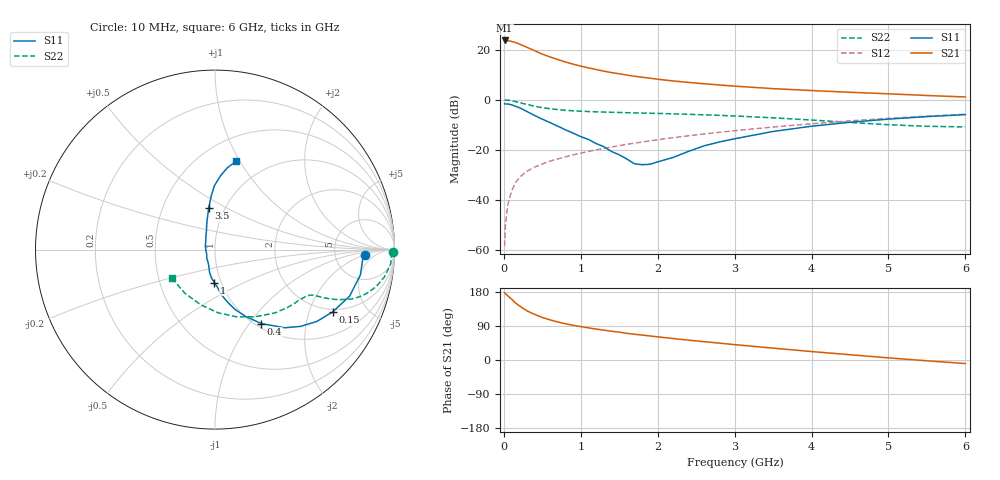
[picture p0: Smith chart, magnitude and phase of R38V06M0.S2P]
! SIEMENS Small Signal Semiconductors
! BFR181
! Si NPN RF Bipolar Junction Transistor in SOT23
! VCE = 8 V  IC = 6 mA
! Common Emitter S-Parameters:  May  1996
# GHz  S  MA  R  50
!  f  S11  S21  S12  S22
! GHz  MAG  ANG  MAG  ANG  MAG  ANG  MAG  ANG
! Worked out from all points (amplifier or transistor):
!   36 points, 10 MHz to 6 GHz, reference 50 ohm
!   highest |S21| = 23.7 dB at 10 MHz (marker M1)
!   |S21| within 3 dB of that: start of sweep to 320.5 MHz
!   unconditionally stable (mu >= 1): 1.124 GHz to 3.021 GHz
!   at 250 MHz: K = 0.45, MSG = 25.6 dB, |S12| = -29.7 dB
!   at 1.4 GHz: K = 1.04, MAG = 13.6 dB, |S12| = -18.9 dB
!   at 6 GHz: K = 0.86, MSG = 3.4 dB, |S12| = -5.8 dB
!   S11 on the Smith chart (normalised r, x): 10 MHz: 11, -2; 150 MHz: 1.88, -2.90; 400 MHz: 1.06, -1.14; 1 GHz: 0.93, -0.35; 3.5 GHz: 0.84, +0.41; 6 GHz: 0.73, +0.96
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0.01  0.8365 -1.9  15.23 177.2  0.0012 86.0  0.9893 -0.9
0.02  0.8248 -3.7  15.18 175.1  0.0031 88.5  0.9833 -1.9
0.05  0.8224 -9.8  15.18 169.7  0.0079 85.3  0.9818 -4.7
0.1  0.7938 -19.0  14.53 160.6  0.015 79.8  0.9567 -9.1
0.15  0.742 -27.9  13.89 150.7  0.022 75.3  0.9209 -13.0
0.2  0.6946 -35.2  12.98 143.2  0.0277 72.7  0.881 -16.0
0.25  0.6397 -42.0  12 136.2  0.0328 70.0  0.8428 -18.3
0.3  0.5833 -48.3  11.13 129.8  0.0375 68.6  0.8065 -20.0
0.4  0.4859 -58.0  9.539 120.4  0.0453 66.2  0.7424 -22.1
0.5  0.4098 -65.3  8.14 112.2  0.0524 65.4  0.6951 -23.2
0.6  0.3503 -71.7  7.144 106.0  0.0598 64.8  0.6627 -23.9
0.7  0.298 -76.8  6.357 100.4  0.066 65.1  0.6365 -24.3
0.8  0.2514 -82.4  5.676 95.7  0.0726 64.8  0.6169 -24.6
1  0.1838 -91.0  4.682 88.1  0.0861 65.4  0.591 -25.4
1.1  0.1616 -96.4  4.329 84.9  0.093 65.6  0.5818 -26.0
1.6  0.0655 -134.6  3.105 70.4  0.129 65.0  0.5519 -30.0
1.8  0.0506 -169.9  2.81 65.8  0.1435 64.6  0.5418 -32.0
2.2  0.0706 136.4  2.372 56.7  0.1752 62.8  0.5231 -36.9
3.5  0.2329 98.7  1.666 31.3  0.2856 53.5  0.4359 -59.1
4.5  0.3553 90.6  1.41 13.9  0.3795 43.3  0.3524 -87.2
5.5  0.4613 81.4  1.215 -2.1  0.4716 31.2  0.2952 -124.9
6  0.5058 76.6  1.136 -9.3  0.5139 24.4  0.2876 -146.3
